PROGRAM MAIN
VAR
	aValues1 : ARRAY [1..2, 1..10] OF INT := [10,20,30,40,50,60,70,80,90,100,100,90,80,70,60,50,40,30,20,10];
	aValues2 : ARRAY [1..10] OF INT := [10,20,30,40,50,60,70,80,90,100];
END_VAR

END_PROGRAM
